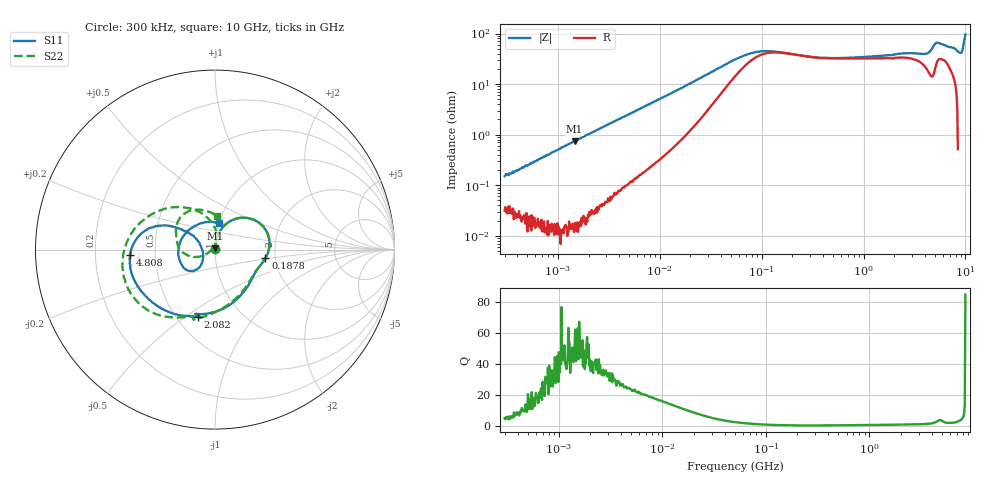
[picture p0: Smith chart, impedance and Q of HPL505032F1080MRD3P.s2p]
! S-Parameter Data Generated by TDK Corporation
! Copyright(C) 2024 TDK Corporation.
! All Rights Reserved.
! TDK P/N: HPL505032F1080MRD3P (SMD / SMT Inductor (Coil))
! Property: L=80nH at 100kHz
! Size(LxWxT): 5x5x3.2mm
! Model Type: s2p (Touchstone File Format Version 1.0)
! Frequency: DC=Yes Start=0.3MHz Stop=10000MHz 802points Log-sweep
! Model Generated on May 28, 2024
! Terms and conditions regarding TDK Simulation Models:
! 1)This simulation model is being provided solely for informational
!  purposes. Please refer to the specifications of the products in
!  terms of detailed characteristics of such products.
! 2)In no event shall TDK Corporation of any of its subsidiaries be
!  liable for any loss or damage arising, directly or indirectly,
!  from any information contained in this simulation model, including,
!  but not limited to loss or damages arising from any inaccuracies,
!  omissions or errors in connection with such information.
! 3)Any and all copyrights on this simulation model are owned by
!  TDK Corporation.  Duplication or redistribution of this simulation
!  model without prior written permission from TDK Corporation
!  is prohibited.
! 4)This simulation model is subject to any modification or change
!  without any prior notice.
! 5)Neither TDK Corporation nor any of its subsidiaries shall make any
!  warranty, express or implied, including but not limited to the
!  correctness, implied warranties of merchantability and fitness for
!  a particular purpose with respect to this simulation models.
! 6)The use of this simulation model shall be deemed to have consented
!  to the terms and conditions hereof.
! Port Assignments:
!  1 ---@@@--- 2
! Applicable Conditions:
!  Temperature = 25 degC
!  DC Bias Current = 0 A
!  Small Signal Operation
# Hz S MA R 50
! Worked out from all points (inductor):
!   801 points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, 300 kHz to 10 GHz, reference 50 ohm
!   read as one part in series: L = 78 nH near 318.3 kHz
!   highest Q = 50.5 at 1.457 MHz (marker M1), where L = 81.1 nH
!   S11 on the Smith chart (normalised r, x): 300 kHz: 1.00, +0.00; 187.8 MHz: 1.77, -0.18; 2.082 GHz: 0.64, -0.56; 4.808 GHz: 0.36, -0.03; 10 GHz: 1.00, +0.30
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300000  0.001484 75.7  0.9998 -0.1  0.9996 -0.1  0.001628 81.3
1456635  0.006881 87.4  0.9998 -0.5  0.9998 -0.5  0.006909 88.8
1713600  0.008133 88.0  0.9997 -0.5  0.9996 -0.5  0.008237 88.4
9671944  0.0454 83.2  0.9958 -3.0  0.9961 -3.0  0.0454 83.2
5.477226e7  0.247 45.9  0.855 -14.6  0.8552 -14.7  0.247 45.9
1.878293e8  0.2853 -9.6  0.7138 -6.8  0.7138 -6.8  0.285 -9.6
3.126428e8  0.2623 -22.7  0.7396 -8.9  0.7396 -8.9  0.2617 -22.7
8.643532e8  0.284 -55.6  0.7178 -25.6  0.718 -25.6  0.2793 -56.7
1.767019e9  0.3606 -97.9  0.6038 -51.0  0.604 -51.0  0.3785 -99.2
2.08171e9  0.3863 -104.2  0.5542 -58.4  0.5544 -58.4  0.3988 -110.3
3.387826e9  0.457 -139.9  0.3404 -85.2  0.3405 -85.2  0.5127 -141.5
4.807583e9  0.4746 -176.6  0.1274 -75.1  0.1273 -75.1  0.5037 179.4
5.364878e9  0.4305 169.9  0.1337 -38.8  0.1337 -38.8  0.4451 160.6
6.41458e9  0.2406 150.0  0.3123 -30.3  0.3127 -30.4  0.259 118.8
6.899057e9  0.1426 147.3  0.4192 -41.4  0.4196 -41.5  0.1545 97.2
7.141296e9  0.09478 156.7  0.4689 -49.1  0.4694 -49.2  0.09907 86.5
7.540283e9  0.07653 -148.8  0.5301 -63.6  0.5306 -63.8  0.01394 120.4
7.875699e9  0.1281 -131.0  0.56 -76.4  0.5601 -76.6  0.07133 -153.0
8.322921e9  0.195 -144.2  0.552 -95.2  0.5516 -95.5  0.1815 -175.0
8.658336e9  0.2053 -160.2  0.5043 -106.4  0.5034 -106.5  0.2245 163.5
9.217363e9  0.1966 163.9  0.418 -122.7  0.4175 -122.7  0.2636 137.3
1e10  0.1488 81.3  0.2773 -125.6  0.2771 -125.6  0.1873 86.9
